PROGRAM MAIN
VAR
	fbSqlDatabase   	 : FB_SQLDatabaseEvt(sNetID := '', tTimeout := T#5S);
	fbSQLStoredProcedure : FB_SQLStoredProcedureEvt(sNetID:='', tTimeout := T#5S);  
	fbSqlResult		     : FB_SQLResultEvt(sNetID:='', tTimeout := T#5S);  
    
	ParaInfo        	 : ST_SQLSPParameter; 
	sRefCursor           : STRING; 
    tcMessage            : I_TcMessage;
	State				 : INT;

	
	fbSqlCommand 		 : FB_SQLCommandEvt(sNetID := '', tTimeout := T#5S);
	
	aRead 				 : ARRAY[0..9] OF ST_StandardRecord;
	
	sCmd: STRING(INT#255);
END_VAR

CASE State OF
	0:
	
	10:  // prepare stored procedure
		(*PostgreSQL Stored Procedure:
		
		CREATE OR REPLACE PROCEDURE "public"."SP_getLastData"(
		    INOUT result_data refcursor)
		LANGUAGE 'plpgsql'
		AS $BODY$
		BEGIN
		    open result_data for SELECT * FROM "myTable_Double" LIMIT 10;
		END
		$BODY$;
		*)
		
		ParaInfo.sParameterName     := '@result_data';
		ParaInfo.eParameterType     := E_SPParameterType.InputOutput;
		ParaInfo.eParameterDataType := E_ColumnType.RefCursor; // 19
		ParaInfo.nParameterSize     := 81;
		
		IF fbSQLDatabase.CreateSP('"public"."SP_getLastData"', ADR(ParaInfo), SIZEOF(ParaInfo), ADR(fbSQLStoredProcedure)) THEN
		    IF fbSQLDatabase.bError THEN
		        State:=255;
		    ELSE
		        State:= State + 1;
		    END_IF
		END_IF
	
	11:  // execute stored procedure
		IF fbSQLStoredProcedure.ExecuteDataReturn(pParameterStrc := ADR(sRefCursor), cbParameterStrc:= SIZEOF(sRefCursor), pSQLDBResult := ADR(fbSqlResult)) THEN
    		IF fbSQLStoredProcedure.bError THEN
    		    tcMessage := fbSQLStoredProcedure.ipTcResult;
    		    State := 255; 
    		ELSE
    		    State := 100; 
    		END_IF    
		END_IF
	
	20:  // PostgreSQL Function
		sCmd := 'SELECT "public"."getLastData"();';
    	
		// call sql command
		IF fbSQLCommand.ExecuteDataReturn(ADR(sCmd), SIZEOF(sCmd), ADR(fbSqlResult)) THEN
		    IF fbSQLCommand.bError THEN
		        tcMessage := fbSQLCommand.ipTcResult;
		        State := 255; // error state
		    ELSE
		        State := 100; 
		    END_IF
		END_IF
		
	100: 
		IF fbSqlResult.Read(0, 10, ADR(aRead), SIZEOF(aRead), TRUE, TRUE) THEN
			IF fbSqlResult.bError THEN
		        tcMessage := fbSqlResult.ipTcResult;
		        State := 255; // error state
		    ELSE
		        State := 0; 
		    END_IF
		END_IF
		
	255: // error handling
		
	
END_CASE

END_PROGRAM
